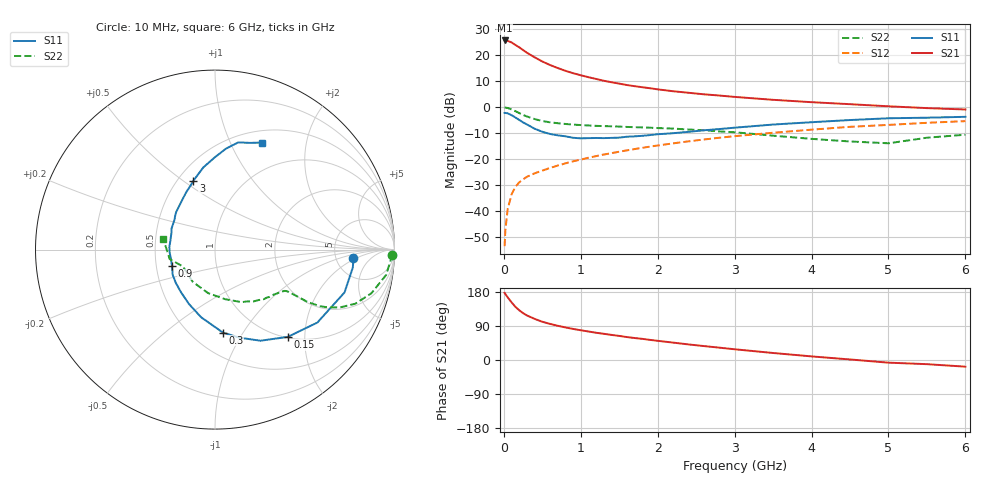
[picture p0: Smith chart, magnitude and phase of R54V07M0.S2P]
! SIEMENS Small Signal Semiconductors
! BFR183
! Si NPN RF Bipolar Junction Transistor in SOT23
! VCE = 4 V  IC = 7 mA
! Common Emitter S-Parameters:  May  1996
# GHz  S  MA  R  50
!  f  S11  S21  S12  S22
! GHz  MAG  ANG  MAG  ANG  MAG  ANG  MAG  ANG
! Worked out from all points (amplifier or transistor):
!   36 points, 10 MHz to 6 GHz, reference 50 ohm
!   highest |S21| = 25.7 dB at 10 MHz (marker M1)
!   |S21| within 3 dB of that: start of sweep to 217.1 MHz
!   unconditionally stable (mu >= 1): 903.7 MHz to 2.571 GHz
!   at 250 MHz: K = 0.52, MSG = 24.9 dB, |S12| = -27.8 dB
!   at 1.4 GHz: K = 1.06, MAG = 12.2 dB, |S12| = -17.7 dB
!   at 6 GHz: K = 0.88, MSG = 2.2 dB, |S12| = -5.4 dB
!   lowest NFmin = 1.25 dB at 450 MHz
!   S11 on the Smith chart (normalised r, x): 10 MHz: 7.38, -1.78; 150 MHz: 1.02, -1.65; 300 MHz: 0.70, -0.82; 900 MHz: 0.60, -0.12; 3 GHz: 0.60, +0.55; 6 GHz: 0.64, +1.32
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0.01  0.7731 -3.6  19.27 177.1  0.0021 90.3  0.9851 -1.6
0.02  0.7744 -7.4  19.01 173.9  0.0043 84.3  0.9805 -3.4
0.05  0.7602 -18.3  18.9 165.4  0.0109 80.6  0.9642 -8.4
0.1  0.7003 -35.5  17.67 152.2  0.0209 73.9  0.9047 -15.6
0.15  0.633 -50.2  15.79 140.4  0.0291 67.9  0.8379 -21.1
0.2  0.5674 -63.5  14.23 131.2  0.0356 64.4  0.7691 -24.7
0.25  0.5086 -74.6  12.59 123.6  0.0407 61.3  0.707 -27.1
0.3  0.4648 -84.5  11.19 117.6  0.0456 60.4  0.6619 -28.4
0.4  0.3847 -101.6  9.132 108.5  0.0531 59.2  0.5904 -29.5
0.5  0.3357 -115.7  7.58 100.9  0.06 59.6  0.5408 -29.6
0.6  0.3042 -128.4  6.491 95.3  0.0673 60.0  0.5103 -29.7
0.7  0.2865 -139.6  5.678 90.3  0.075 60.8  0.4914 -29.8
0.9  0.2571 -158.9  4.51 82.0  0.0905 61.6  0.4615 -30.1
1.1  0.2531 -176.0  3.78 75.2  0.1062 62.2  0.4444 -31.5
1.3  0.2533 170.7  3.226 69.1  0.1224 62.1  0.4313 -33.0
1.6  0.2695 153.7  2.668 60.5  0.1472 61.2  0.4161 -36.6
2.2  0.315 129.1  2.027 45.9  0.2006 57.9  0.3867 -45.7
3  0.4024 107.4  1.576 28.3  0.2764 50.4  0.3284 -63.1
3.5  0.4625 98.1  1.385 18.5  0.3215 44.6  0.2822 -78.4
4.5  0.5648 83.9  1.141 1.4  0.418 32.6  0.2183 -124.6
5.5  0.6266 71.6  0.959 -11.0  0.4995 20.5  0.2579 -168.2
6  0.6516 66.3  0.902 -17.6  0.5381 12.6  0.2947 168.1
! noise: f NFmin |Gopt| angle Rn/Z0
0.45  1.25  0.18  42  0.22
0.9  1.3  0.22  110  0.2
1.8  2  0.33  180  0.14
